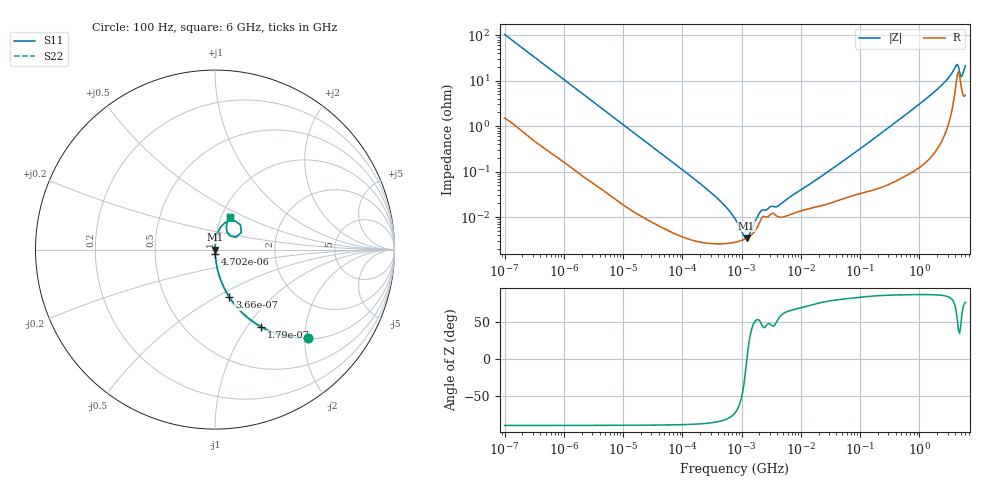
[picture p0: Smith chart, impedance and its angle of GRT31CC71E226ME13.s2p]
!Murata Part Number: GRT31CC71E226ME13
!These Parameters are Measured in Series Mode Connection
!Data Generated on Jun 19, 2026
!  o--ll--o
!Port1  Port2
!  o------o
!Operation Temp=25[degC], DC Bias Voltage=0[V]
!Freq. Start=100[Hz] Stop=6[GHz] 401[Steps]
# Hz S RI R 50
!Freq.(Hz) S11(Real) S11(Imag) S21(Real) S21(Imag) S12(Real) S12(Imag) S22(Real) S22(Imag)
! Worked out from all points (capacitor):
!   401 points, 100 Hz to 6 GHz, reference 50 ohm
!   read as one part in series: C = 15.3 uF near 109 Hz
!   lowest |Z| = 3.46 mohm at 1.212 MHz (marker M1)
!   series resonance near 1.228 MHz, so ESL is about 1.1 nH
!   S11 on the Smith chart (normalised r, x): 100 Hz: 1.03, -2.07; 179 Hz: 1.02, -1.17; 366 Hz: 1.01, -0.57; 4.702 kHz: 1.00, -0.05; 6 GHz: 1.10, +0.42
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100  0.5175 -0.4925  0.4825 0.4925  0.4825 0.4925  0.5175 -0.4925
179  0.2568 -0.4295  0.7432 0.4295  0.7432 0.4295  0.2568 -0.4295
366  0.0791 -0.2628  0.9209 0.2628  0.9209 0.2628  0.0791 -0.2628
784  0.0198 -0.1319  0.9802 0.1319  0.9802 0.1319  0.0198 -0.1319
2008  0.00363 -0.0529  0.9964 0.0529  0.9964 0.0529  0.00363 -0.0529
4702  0.000902 -0.0229  0.9991 0.0229  0.9991 0.0229  0.000902 -0.0229
40335  7.11e-05 -0.00272  0.9999 0.00272  0.9999 0.00272  7.11e-05 -0.00272
289253  2.64e-05 -0.000365  1 0.000365  1 0.000365  2.64e-05 -0.000365
774597  2.8e-05 -8.77e-05  1 8.77e-05  1 8.77e-05  2.8e-05 -8.77e-05
1212075  3.45e-05 -2.4e-06  1 2.4e-06  1 2.4e-06  3.45e-05 -2.4e-06
1734173  5.24e-05 6.86e-05  0.9999 -6.86e-05  0.9999 -6.86e-05  5.24e-05 6.86e-05
2268635  0.000102 0.000101  0.9999 -0.000101  0.9999 -0.000101  0.000102 0.000101
3103719  0.000116 0.000125  0.9999 -0.000125  0.9999 -0.000125  0.000116 0.000125
4060267  0.000103 0.000139  0.9999 -0.000139  0.9999 -0.000139  0.000103 0.000139
1.555665e7  0.000159 0.000553  0.9998 -0.000553  0.9998 -0.000553  0.000159 0.000553
3.124326e8  0.00062 0.00954  0.9994 -0.00954  0.9994 -0.00954  0.00062 0.00954
1.95892e9  0.00685 0.062  0.9931 -0.062  0.9931 -0.062  0.00685 0.062
3.205649e9  0.0264 0.1161  0.9736 -0.1161  0.9736 -0.1161  0.0264 0.1161
4.009986e9  0.0823 0.1605  0.9177 -0.1605  0.9177 -0.1605  0.0823 0.1605
4.385646e9  0.1415 0.1385  0.8585 -0.1385  0.8585 -0.1385  0.1415 0.1385
5.245841e9  0.0675 0.0978  0.9325 -0.0978  0.9325 -0.0978  0.0675 0.0978
6e9  0.0816 0.1821  0.9184 -0.1821  0.9184 -0.1821  0.0816 0.1821
